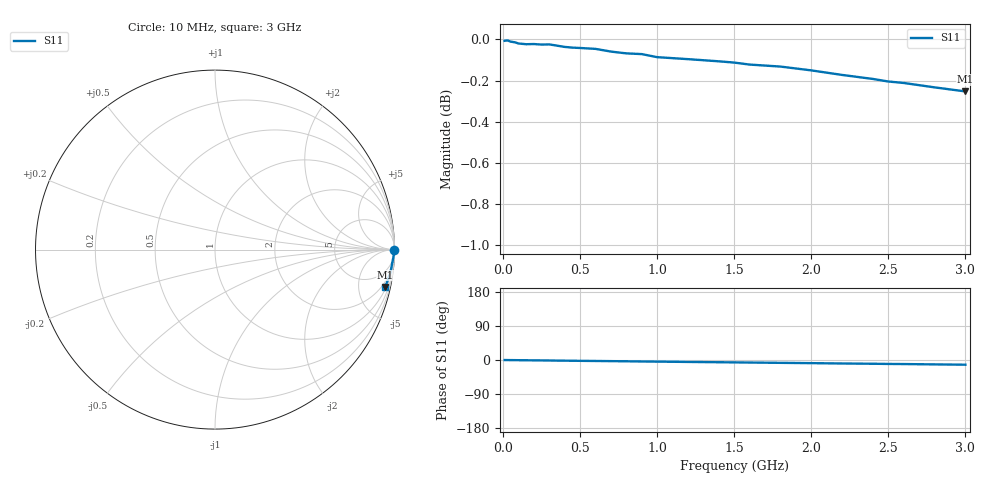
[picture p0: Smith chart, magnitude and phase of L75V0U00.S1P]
! SIEMENS Small Signal Semiconductors
! BAR14-1
! Si PIN Diode in SOT23
! VR = 5 V
! S-Parameters:  July  1992
# GHz  S  MA  R  50
!  f  S11
! GHz  MAG  ANG
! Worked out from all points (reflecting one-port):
!   31 points, 10 MHz to 3 GHz, reference 50 ohm
!   lowest |S11| = -0.3 dB at 3 GHz (marker M1), VSWR 68.69, Z = 61.3 - j452 ohm
!   phase of S11 starts at -0 deg and turns -12 deg over the sweep
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0.01  0.9992 -0.1
0.03  0.9994 -0.2
0.05  0.9987 -0.3
0.06  0.9986 -0.3
0.08  0.9983 -0.4
0.1  0.9977 -0.5
0.15  0.9973 -0.7
0.2  0.9974 -0.9
0.25  0.9971 -1.1
0.3  0.9972 -1.3
0.35  0.9965 -1.6
0.4  0.9958 -1.8
0.6  0.9947 -2.6
0.7  0.9932 -3.0
0.8  0.9922 -3.4
0.9  0.9918 -3.9
1  0.9901 -4.3
1.2  0.989 -5.1
1.5  0.9871 -6.3
1.6  0.986 -6.7
1.8  0.9849 -7.5
2  0.9828 -8.3
2.2  0.9803 -9.2
2.4  0.9781 -9.9
2.5  0.9767 -10.4
2.6  0.9759 -10.7
2.8  0.9735 -11.6
3  0.9713 -12.4
